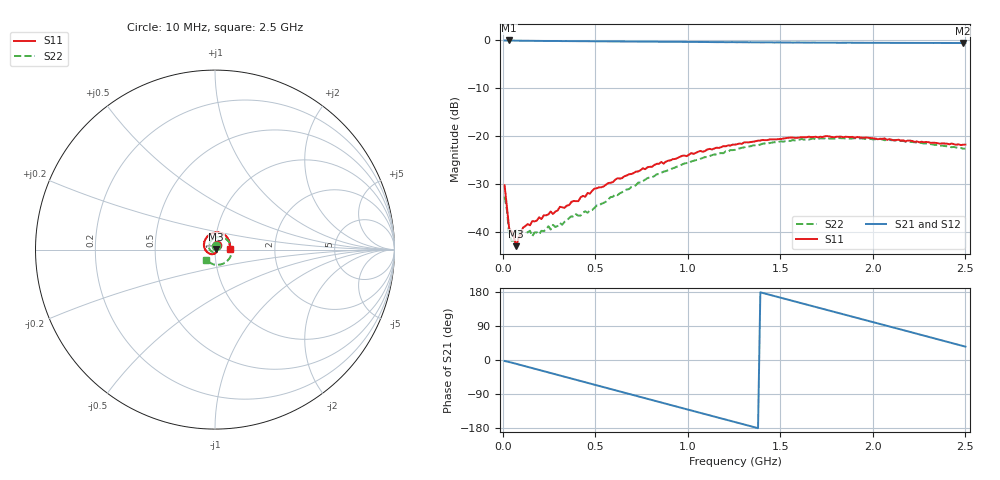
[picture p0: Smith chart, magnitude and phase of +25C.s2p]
!Agilent Technologies,E8364B,MY43040864,A.07.50.48
!Agilent E8364B: A.07.50.48
!Date: Tuesday, September 09, 2025 17:15:16
!Correction: S11(Full 2 Port(1,2))
!S21(Full 2 Port(1,2))
!S12(Full 2 Port(1,2))
!S22(Full 2 Port(1,2))
!S2P File: Measurements: S11, S21, S12, S22:
# Hz S  dB  R 50
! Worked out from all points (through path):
!   201 points, 10 MHz to 2.5 GHz, reference 50 ohm
!   highest |S21| = -0.04 dB at 34.9 MHz (marker M1); lowest = -0.6 dB at 2.488 GHz (marker M2)
!   group delay of S21, straight-line fit = 360 ps
!   lowest |S11| = -43.0 dB at 72.25 MHz (marker M3), VSWR 1.01, Z = 50.7 + j0.174 ohm
!   |S11| at or under -10 dB: start of sweep to end of sweep
!   |S22| runs from -41.9 to -20.4 dB; largest |S21 - S12| = 0.0055
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1e7  -30.31 68.0  -0.05 -2.7  -0.02 -2.9  -32.67 69.2
2.245e7  -34.75 59.0  -0.05 -4.0  -0.05 -4.0  -35.47 67.1
3.49e7  -39.37 48.4  -0.04 -5.2  -0.03 -5.1  -40.68 52.4
5.98e7  -40.93 29.8  -0.06 -8.4  -0.07 -8.4  -41.89 31.4
7.225e7  -43.02 14.1  -0.08 -10.0  -0.07 -9.9  -39.71 21.3
1.096e8  -39.13 9.6  -0.10 -14.9  -0.09 -14.9  -40.02 15.2
1.9675e8  -36.99 -35.5  -0.13 -26.3  -0.12 -26.2  -40.53 -37.9
2.4655e8  -36.39 -52.4  -0.14 -32.7  -0.13 -32.7  -38.85 -52.2
2.59e8  -35.77 -53.4  -0.14 -34.4  -0.13 -34.4  -39.54 -60.2
2.7145e8  -36.29 -54.3  -0.15 -36.0  -0.14 -36.0  -38.57 -64.5
4.333e8  -32.52 -100.4  -0.19 -57.1  -0.19 -57.0  -36.01 -110.6
6.325e8  -28.91 -138.6  -0.25 -83.0  -0.24 -83.1  -31.97 -167.4
8.4415e8  -25.79 -172.9  -0.30 -110.5  -0.30 -110.5  -27.96 146.5
1.0807e9  -23.29 150.0  -0.36 -141.2  -0.35 -141.2  -24.59 104.9
1.255e9  -21.81 126.0  -0.40 -163.8  -0.40 -163.8  -22.90 74.9
1.4542e9  -20.72 101.3  -0.43 170.5  -0.46 170.6  -21.40 42.6
1.6783e9  -20.21 73.3  -0.47 141.7  -0.49 141.7  -20.50 6.8
1.8775e9  -20.23 51.7  -0.51 115.9  -0.50 115.9  -20.54 -24.2
2.08915e9  -20.65 31.8  -0.54 88.5  -0.53 88.6  -20.84 -58.6
2.2759e9  -21.32 16.8  -0.55 64.4  -0.54 64.3  -21.57 -90.2
2.48755e9  -21.83 4.5  -0.58 36.9  -0.57 36.8  -22.65 -127.4
2.5e9  -21.80 3.2  -0.58 35.3  -0.58 35.2  -22.65 -130.3
